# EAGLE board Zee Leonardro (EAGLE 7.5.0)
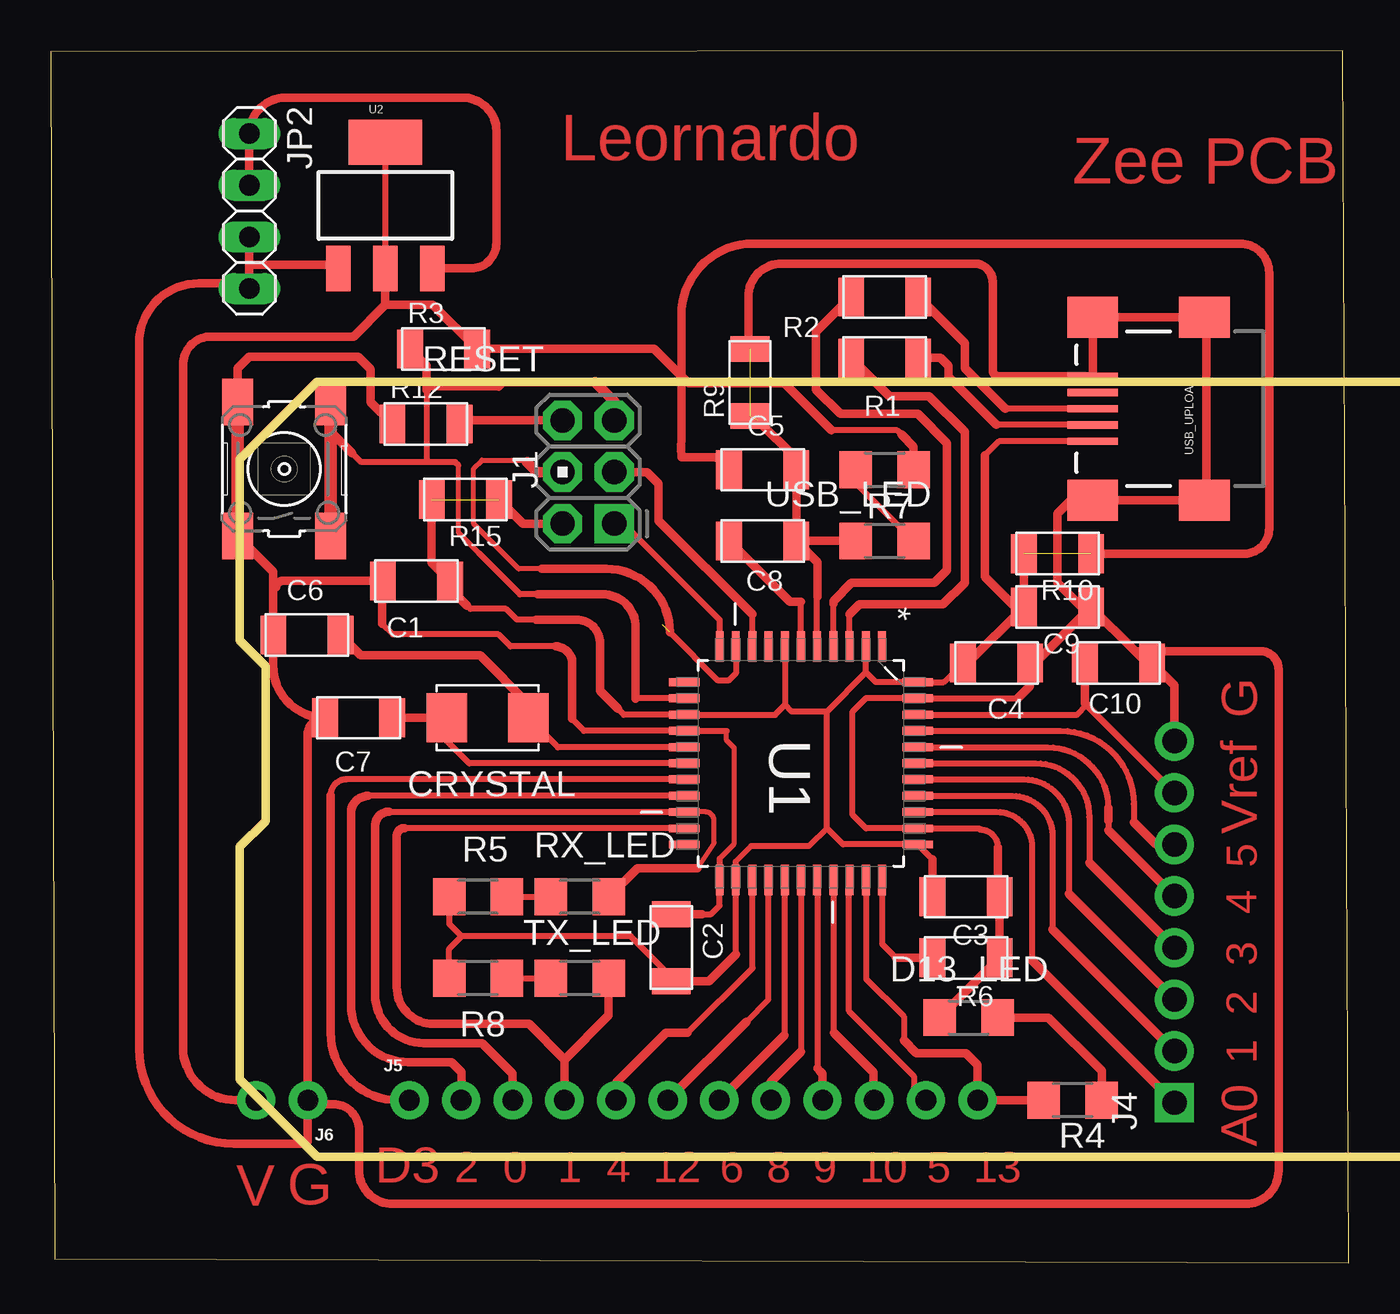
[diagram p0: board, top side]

Size 63.84 x 59.6 mm. Coordinates in mm from the lower left corner, seen from the top.
Outline: 0.19,0.21 63.84,0 63.56,59.6 0,59.57 0.19,0.21
Copper layers (1*16): Top 0.035mm / dielectric 1.5mm / Bottom 0.035mm
Design rules "default *": minimum track width 10mil, minimum drill 24mil, track to track 0.4mm, track to pad 0.4mm, pad to pad 0.4mm, via to via 0.4mm, smd to smd 0.4mm, copper to edge 40mil, drill to drill 0.4mm, minimum pad ring 10mil, minimum via ring 8mil, stop-mask expansion 4mil, vias tented up to drill 0mil, thermal gap 10mil
Net classes: 0 default: width 0.305 mm, drill 0.305 mm, clearance 0.305 mm
Milling: area 9.3,5.2 to 109.6,43.3

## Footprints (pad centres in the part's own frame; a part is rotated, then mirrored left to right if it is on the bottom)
C1206FAB = smd 1.27 x 1.905: 1 -1.651,0; 2 1.651,0
2-SMD-5X3MM = smd 2 x 2.4: P$1 -2,0; P$2 2,0
1206 = smd 1.6 x 1.803: 1 -1.422,0; 2 1.422,0
2X3-NS = drill 1.2 pad 1.93 square: 1 -2.54,-1.27 | drill 1.2 pad 1.93 octagon: 2 -2.54,1.27; 3 0,-1.27; 4 0,1.27; 5 2.54,-1.27; 6 2.54,1.27
1X08_PIN1_NO_SILK = drill 1.2 pad 1.93 square: 1 0,0 | drill 1.2 pad 1.93: 2 2.54,0; 3 5.08,0; 4 7.62,0; 5 10.16,0; 6 12.7,0; 7 15.24,0; 8 17.78,0
1X12_NO_SILK = drill 1.016 pad 1.88: 1 0,0; 2 2.54,0; 3 5.08,0; 4 7.62,0; 5 10.16,0; 6 12.7,0; 7 15.24,0; 8 17.78,0; 9 20.32,0; 10 22.86,0; 11 25.4,0; 12 27.94,0
1X02_NO_SILK = drill 1.016 pad 1.88: 1 0,0; 2 2.54,0
1X04 = drill 1.016 long: 1 -3.81,0; 2 -1.27,0; 3 1.27,0; 4 3.81,0
R1206FAB = smd 1.27 x 1.905: 1 -1.651,0; 2 1.651,0
6MM_SWITCH = smd 2.286 x 1.524: 1 -3.302,2.286; 2 3.302,2.286; 3 -3.302,-2.286; 4 3.302,-2.286
QFP80P1200X1200X120-44N = smd 1.5 x 0.38: 1 -5.74,3.988; 2 -5.74,3.2; 3 -5.74,2.388; 4 -5.74,1.6; 5 -5.74,0.787; 6 -5.74,0; 7 -5.74,-0.787; 8 -5.74,-1.6; 9 -5.74,-2.388; 10 -5.74,-3.2; 11 -5.74,-3.988; 23 5.74,-3.988; 24 5.74,-3.2; 25 5.74,-2.388; 26 5.74,-1.6; 27 5.74,-0.787; 28 5.74,0; 29 5.74,0.787; 30 5.74,1.6; 31 5.74,2.388; 32 5.74,3.2; 33 5.74,3.988 | smd 0.38 x 1.5: 12 -3.988,-5.74; 13 -3.2,-5.74; 14 -2.388,-5.74; 15 -1.6,-5.74; 16 -0.787,-5.74; 17 0,-5.74; 18 0.787,-5.74; 19 1.6,-5.74; 20 2.388,-5.74; 21 3.2,-5.74; 22 3.988,-5.74; 34 3.988,5.74; 35 3.2,5.74; 36 2.388,5.74; 37 1.6,5.74; 38 0.787,5.74; 39 0,5.74; 40 -0.787,5.74; 41 -1.6,5.74; 42 -2.388,5.74; 43 -3.2,5.74; 44 -3.988,5.74
SOT223 = smd 1.219 x 2.235: 1 -2.311,-3.099; 2 0,-3.099; 3 2.311,-3.099 | smd 3.6 x 2.2: 4 0,3.099
USB_MINIB = smd 2.5 x 0.35: D+ 3.77,0; D- 3.77,0.8; GND 3.77,-1.6; ID 3.77,-0.8; VBUS 3.77,1.6 | smd 2.5 x 2: SHIELD@1 -1.73,-4.5; SHIELD@2 -1.73,4.5; SHIELD@3 3.77,4.5; SHIELD@4 3.77,-4.5

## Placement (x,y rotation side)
C1  0.1uF  [C1206FAB]  17.98,33.54 180 top
C2  0.1uF  [C1206FAB]  30.52,15.5 90 top
C3  0.1uF  [C1206FAB]  45.02,18 0 top
C4  0.1uF  [C1206FAB]  46.52,29.5 0 top
C5  0.1uF  [C1206FAB]  35.02,39 0 top
C6  18pF  [C1206FAB]  12.6,30.87 180 top
C7  18pF  [C1206FAB]  15.14,26.81 180 top
C8  0.1uF  [C1206FAB]  35.02,35.5 0 top
C9  0.1uF  [C1206FAB]  49.52,32.25 0 top
C10  0.1uF  [C1206FAB]  52.52,29.5 0 top
CRYSTAL  CRYSTAL  [2-SMD-5X3MM]  21.49,26.81 0 top
D13_LED  [1206]  45.14,12.06 180 top
J1  AVR_SPI_PRG_6NS  [2X3-NS]  26.44,38.89 90 top
J4  [1X08_PIN1_NO_SILK]  55.27,7.88 90 top
J5  [1X12_NO_SILK]  17.64,8 0 top
J6  [1X02_NO_SILK]  12.64,8 180 top
JP2  [1X04]  9.77,51.72 270 top
R1  22  [R1206FAB]  41.02,44.5 0 top
R2  22  [R1206FAB]  41.02,47.5 0 top
R3  10K  [R1206FAB]  19.32,44.94 0 top
R4  499  [1206]  50.27,8 0 top
R5  499  [1206]  21.02,18 0 top
R6  680  [R1206FAB]  45.02,15 0 top
R7  499  [1206]  41.02,39 180 top
R8  499  [1206]  21.02,14 0 top
R9  0  [R1206FAB]  34.39,43.29 90 top
R10  0  [R1206FAB]  49.52,34.88 180 top
R12  0  [R1206FAB]  18.45,41.25 0 top
R15  0  [R1206FAB]  20.39,37.53 180 top
RESET  [6MM_SWITCH]  11.48,39.04 90 top
RX_LED  [1206]  26.02,18 0 top
TX_LED  [1206]  26.02,14 0 top
U1  ATMEGA32U4-AU  [QFP80P1200X1200X120-44N]  36.9,24.57 270 top
U2  [SOT223]  16.45,52 0 top
USB_LED  [1206]  41.02,35.5 180 top
USB_UPLOAD  USB_MINIB  [USB_MINIB]  55.02,42 180 top

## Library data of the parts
C1-C10 CRYSTAL R1-R3 R6 R9 R10 R12 R15 RESET USB_UPLOAD = fab
D13_LED R4 R5 R7 R8 RX_LED TX_LED USB_LED = ng
J1 J4 = SparkFun-ConnectorsModified
J5 J6 = SparkFun-Connectors
JP2 = pinhead
U1 = Atmel_By_element14_Batch_1; MPN: ATMEGA32U4-AU; OC_FARNELL: 1748525; OC_NEWARK: 26R5633; PACKAGE: TQFP-44; SUPPLIER: Atmel
U2 = fab; PROD_ID: VREG-08170

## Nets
12V: JP2.1 JP2.2 U2.3
A0: J4.1 U1.36
A1: J4.2 U1.37
A2: J4.3 U1.38
A3: J4.4 U1.39
A4: J4.5 U1.40
A5: J4.6 U1.41
AREF: C10.1 J4.7 U1.42
D0: J5.3 RX_LED.2 U1.20
D1: J5.4 TX_LED.2 U1.21
D2: J5.2 U1.19
D3: J5.1 U1.18
D4: J5.5 U1.25
D5: J5.11 U1.31
D6: J5.7 U1.27
D7: U1.1
D8: J5.8 U1.28
D9: J5.9 U1.29
D10: J5.10 U1.30
D11: U1.12
D12: J5.6 U1.26
D13: J5.12 R4.1 U1.32
D14: U1.8
D15: J1.3 U1.9
D16: J1.4 U1.10
D17: J1.1 U1.11
D+: R2.1 U1.4
D-: R1.1 U1.3
GND: C1.2 C2.2 C3.2 C4.2 C5.2 C6.2 C7.2 C8.2 C9.2 C10.2 D13_LED.2 J4.8 J6.1 JP2.3 JP2.4 R6.2 R9.1 R9.2 R12.1 RESET.1 RESET.2 U1.5 U1.15 U1.23 U1.35 U1.43 U2.1 USB_LED.2 USB_UPLOAD.GND USB_UPLOAD.SHIELD@1 USB_UPLOAD.SHIELD@2 USB_UPLOAD.SHIELD@3 USB_UPLOAD.SHIELD@4
N$1: R1.2 USB_UPLOAD.D-
N$2: R2.2 USB_UPLOAD.D+
N$3: D13_LED.1 R4.2
N$4: R5.2 RX_LED.1
N$5: R7.2 USB_LED.1
N$6: R8.2 TX_LED.1
N$13: J1.6 R12.2
N$35: R6.1 U1.33
RESET: J1.5 R3.1 RESET.3 RESET.4 U1.13
TXLED: U1.22
UCAP: C8.1 U1.6
VCC: C1.1 C2.1 C3.1 C4.1 C5.1 C9.1 J1.2 J6.2 R3.2 R5.1 R7.1 R8.1 R10.1 R10.2 R15.1 R15.2 U1.2 U1.7 U1.14 U1.24 U1.34 U1.44 U2.2 U2.4 USB_UPLOAD.VBUS
XTAL1: C7.1 CRYSTAL.P$1 U1.17
XTAL2: C6.1 CRYSTAL.P$2 U1.16

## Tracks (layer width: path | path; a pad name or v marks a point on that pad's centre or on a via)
12V
  Top 0.406: JP2.2 JP2.1 arc-90 11.52,57.29 19.53,57.29 20.29,57.29 | 20.29,57.29 20.55,57.29 | U2.3 arc90 18.57,48.7 18.57,48.37 arc-90 19.1,48.91 20.67,48.91 arc90 21.92,50.15 21.92,55.66 arc90 20.29,57.29
A0
  Top 0.305: U1.36 46.53,22.18 arc-90 48.27,20.44 48.27,14.88
  Top 0.406: 48.27,14.88 J4.1
A1
  Top 0.305: U1.37 47.3,22.97 arc-90 49.27,21 49.27,16.42
  Top 0.406: 49.27,16.42 J4.2
A2
  Top 0.305: U1.38 47.86,23.78 arc-90 50.08,21.56 50.08,18.14
  Top 0.406: 50.08,18.14 J4.3
A3
  Top 0.305: U1.39 48.45,24.57 arc-90 51.08,21.94 51.08,19.68
  Top 0.406: 51.08,19.68 J4.4
A4
  Top 0.305: U1.40 49.04,25.35 arc-90 52.02,22.38 | 52.02,21.75 52.02,21.29
  Top 0.406: 52.02,21.29 J4.5 | 52.02,22.38 52.02,21.75
A5
  Top 0.305: U1.41 49.68,26.17 arc-90 53.27,22.58 53.27,21.66
  Top 0.406: 53.27,21.66 54.35,20.58 J4.6
AREF
  Top 0.305: U1.42 50.47,26.95 50.95,27.43
  Top 0.356: 50.95,27.43 J4.7
  Top 0.406: 50.95,27.43 50.86,27.52 C10.1
D0
  Top 0.254: 31.8,19.42 32.64,20.66 arc-90 32.61,20.69 32.61,21.78 arc90 32.21,22.18 U1.20
  Top 0.305: 16.64,22.19 U1.20
  Top 0.406: 22.77,8 J5.3 22.7,8.02 22.7,9.31 21.2,10.81 18.33,10.81 arc-90 15.95,13.19 15.95,21.5 arc-90 16.64,22.19 | RX_LED.2 28.85,19.42 31.8,19.42
D1
  Top 0.305: 17.39,21.38 17.4,21.37 U1.21
  Top 0.406: 25.27,10 23.52,11.75 19.33,11.75 18.83,11.75 arc-90 17.02,13.56 17.02,21 arc-90 17.39,21.38 | 25.27,10 J5.4 | TX_LED.2 27.44,12.17 25.27,10
D2
  Top 0.305: U1.19 15.61,22.97
  Top 0.406: J5.2 20.2,8.02 20.2,9.38 19.7,9.88 18.08,9.88 17.58,9.88 arc-90 14.77,12.69 14.77,22.13 arc-90 15.61,22.97
D3
  Top 0.305: U1.18 14.54,23.78 arc90 13.77,23
  Top 0.406: 13.77,23 13.77,11.88 arc90 13.76,11.88 13.76,11.31 arc90 17.08,8 J5.1
D4
  Top 0.305: U1.25 34.52,14.5 31.33,11.31
  Top 0.406: J5.5 27.8,8.85 30.27,11.31 31.33,11.31
D5
  Top 0.305: U1.31 39.27,18.81 39.27,12.38 42.45,9.19 42.45,8.59 J5.11
D6
  Top 0.305: U1.27 36.08,18.8 36.08,11.19
  Top 0.406: J5.7 35.5,10.61 36.08,11.19
D8
  Top 0.305: 36.89,10.38 36.9,10.38 U1.28
  Top 0.406: 36.89,10.38 35.39,8.88 35.39,8.03 J5.8
D9
  Top 0.305: U1.29 37.7,18.81 37.7,9.56
  Top 0.406: J5.9 37.96,9.31 37.84,9.42 37.7,9.56
D10
  Top 0.305: 38.78,11.05 38.5,11.33 U1.30
  Top 0.406: 38.52,11.31 38.78,11.05 40.45,9.38 40.45,8.05 J5.10
D12
  Top 0.305: U1.26 35.3,12.96 34.21,11.87
  Top 0.406: J5.6 34.21,11.87
D13
  Top 0.305: 41.95,10.94 41.95,12.13 40.1,13.98 U1.32
  Top 0.406: R4.1 J5.12 45.58,9.75 45.02,10.31 42.58,10.31 41.95,10.94
D15
  Top 0.305: U1.9 34.51,31.88
  Top 0.406: J1.3 29.32,38.89 29.89,38.31 29.89,36.5 34.51,31.88
D16  (1 unrouted)
  Top 0.254: 24.14,34.13 23.02,34.13 20.8,36.35 20.8,39.06 21.2,39.47 23.33,39.47 23.42,39.38 23.55,39.25
  Top 0.305: U1.10 33.7,28.99 33.33,28.63 32.83,28.63 30.45,31
  Top 0.406: 24.14,34.13 27.33,34.13 arc-90 30.45,31
  Top 0.508: J1.4 23.91,38.89 23.42,39.38
D17
  Top 0.305: U1.11 32.91,31.61 28.17,36.35 J1.1
D+
  Top 0.305: U1.4 38.5,32.42
  Top 0.406: 38.5,32.42 38.5,32.54 39.39,33.44 43.45,33.44 44.08,34.06 44.08,40.31 42.64,41.75 38.83,41.75 37.64,42.94 37.64,45.78 R2.1
D-
  Top 0.305: U1.3 39.28,31.89
  Top 0.406: R1.1 41.24,42.63 43.2,42.63 44.95,40.88 44.95,33.44 43.89,32.38 39.77,32.38 39.28,31.89
GND  (2 unrouted)
  Top 0.254: 32.91,19.89 33.63,20.61 33.63,25.31 33.24,25.69 33.24,26.15
  Top 0.305: U1.5 37.68,32.73 37.7,32.75 | 25.64,26.75 26.23,26.17 U1.15 33.24,26.17 33.24,26.15 | RESET.1 9.71,35.22 | 47.58,27.77 U1.43 40.1,27.77 39.44,27.11 39.44,22.03 40.1,21.37 U1.35 45.65,21.37 45.7,21.31 arc-90 46.58,20.44 | 32.04,17.15 32.48,17.15 32.89,17.56 32.89,18.81 U1.23 32.91,19.89 | 24.83,30.31 22.61,30.31 22.02,30.91 16.83,30.91 16.3,31.44 | 50.86,32.1 50.67,32.28
  Top 0.406: 46.58,20.44 46.58,18.09 C3.2 R6.2 D13_LED.2 | 56.58,37.5 USB_UPLOAD.SHIELD@3 50.17,37.5 49.52,36.85 49.52,33.44 50.67,32.28 50.93,32.02 | 56.58,37.5 USB_UPLOAD.SHIELD@2 | RESET.2 9.19,44 9.76,44.56 15.11,44.56 15.73,43.94 15.73,42.32 R12.1 | C2.2 32.04,17.15 | 37.7,32.75 37.7,34.47 C8.2 | C8.2 USB_LED.2 | C8.2 C5.2 36.67,39.54 34.77,41.44 | 25.64,26.75 25.64,29.5 arc90 24.83,30.31 | J4.8 55.27,28.4 C10.2 53.92,29.5 53.33,30.09 | 53.33,30.09 C9.2 50.93,32.02 | 50.93,32.02 48.42,29.5 C4.2 48.17,28.36 47.58,27.77 | 12.7,7.94 J6.1 | 56.58,37.5 56.83,37.75 56.83,46.42 USB_UPLOAD.SHIELD@1 USB_UPLOAD.SHIELD@4 USB_UPLOAD.GND 46.63,43.6 arc-90 46.33,43.9 46.33,48.25 arc90 45.44,49.14 35.94,49.14 arc90 34.31,47.51 34.31,45.02 arc90 R9.2 34.83,44.94 | 16.3,31.44 16.3,33.5 C1.2 11.4,33.54 arc90 11.08,33.22 10.95,33.22 | J6.1 12.99,7.66 arc-90 13.14,7.81 13.89,7.81 arc-90 15.16,6.54 15.16,4.56 arc90 16.81,2.91 58.77,2.91 arc90 60.39,4.53 60.39,29.18 arc90 59.48,30.09 53.33,30.09 | 10.95,33.22 C6.2 10.95,29.35 arc90 C7.2 C7.2 arc90 12.64,25.96 J6.1 | 10.95,33.22 10.95,33.99 9.71,35.22 | 9.77,49.08 JP2.4 arc90 9.51,48.17 7.29,48.17 arc90 4.34,45.22 4.34,10.53 arc90 9.02,5.85 12.44,5.85 arc90 12.64,6.05 J6.1 | 9.77,49.08 JP2.3 | U2.1 14.14,49.08 9.77,49.08
  Top 0.61: RESET.1 RESET.2
N$1
  Top 0.305: USB_UPLOAD.D- 46.5,41.2
  Top 0.406: 46.5,41.2 44.14,43.56 44.14,44.13 43.77,44.5 R1.2
N$2
  Top 0.305: USB_UPLOAD.D+ 46.95,42
  Top 0.406: 46.95,42 44.95,44 44.95,45.22 R2.2
N$3
  Top 0.406: R4.2 51.69,9.46 49.08,12.06 D13_LED.1
N$4
  Top 0.305: R5.2 RX_LED.1
N$5
  Top 0.305: R7.2 39.59,38.35 USB_LED.1
N$6
  Top 0.305: R8.2 TX_LED.1
N$13
  Top 0.406: R12.2 20.29,41.44 25.16,41.44
  Top 0.508: 25.16,41.44 J1.6
N$35
  Top 0.305: U1.33 40.88,16.28 40.88,15.88 40.88,15.7 41.58,15
  Top 0.406: 41.58,15 R6.1
RESET
  Top 0.254: 21.05,34.91 20.05,35.91 20.05,39.22
  Top 0.305: U1.13 28.78,27.77 28.77,27.75 | 23.95,32.88 23.08,32.88 21.05,34.91 | 20.05,39.22 19.89,39.38 18.48,39.38 | 18.48,39.38 15.27,39.38 14.83,39.81 | 18.48,42.91 18.48,39.38 | 22.33,43.31 22.05,43.03 18.55,43.03 18.48,43.1
  Top 0.406: RESET.4 13.76,40.88 14.83,39.81 | 28.77,27.75 28.77,31.25 arc90 27.14,32.88 23.95,32.88 | 26.77,43.31 22.33,43.31 | R3.1 18.48,44.12 18.48,43.1 18.48,42.91
  Top 0.508: J1.5 27.71,42.37 26.77,43.31
  Top 0.61: RESET.4 RESET.3
UCAP
  Top 0.305: U1.6 36.9,32.5 36.89,32.5
  Top 0.406: 36.89,32.5 36.36,32.5 C8.1
VCC  (2 unrouted)
  Top 0.254: 33.7,19.74 34.45,20.5
  Top 0.305: 38.17,21.38 38.17,27.11 | U1.7 36.11,27.44 | 40.1,29.04 40.58,28.56 U1.44 43.92,28.56 C4.1 | 40.1,29.04 38.17,27.11 | 36.11,27.44 35.62,26.95 U1.14 28.19,26.95 27.89,27.25 | 38.17,27.11 36.44,27.11 36.11,27.44 | 38.17,21.38 38.96,20.58 U1.34 43.36,19.85 | 38.17,21.38 37.29,20.5 34.45,20.5 | 40.1,29.04 U1.2 | 33.7,15.19 U1.24 33.7,19.74 | C2.1 30.52,14.06 28.52,16.06 20.2,16.06 | R5.1 19.59,16.67 20.2,16.06 | R8.1 19.59,15.46 20.2,16.06 | 41.83,40.75 41.64,40.94 38.39,40.94 | USB_UPLOAD.VBUS 46.64,40.4 45.95,39.71 | 20.48,32.31 20.64,32.16 22.39,32.16 22.92,31.63 23.86,31.63 24.02,31.63 | U2.4 U2.2
  Top 0.406: C2.1 32.36,13.85 33.7,15.19 | R7.1 42.44,40.14 41.83,40.75 | 38.39,40.94 36.08,43.25 31.36,43.25 31.02,43.6 | C4.1 45.11,29.5 C9.1 | 47.79,32.33 C9.1 | C9.1 48.02,32.4 47.86,32.55 R10.2 | 10.2,8 J6.2 9.1,8 arc-90 6.5,10.6 6.5,44.16 arc-90 7.9,45.55 14.88,45.55 16.45,47.12 | C9.1 47.45,32.25 45.95,33.75 45.95,39.71 | C3.1 43.36,19.85 | C1.1 | 20.48,32.31 19.64,33.16 C1.1 | R15.1 23.23,36.35 J1.2 | R15.2 18.74,34.43 C1.1 | 31.02,43.6 31.02,40.58 30.99,40.09 31.02,39.63 32.53,39.63 arc-90 33.26,38.9 arc90 C5.1 | 31.02,43.6 29.67,44.94 R3.2 18.79,47.12 16.45,47.12 | 27.89,27.25 27.02,28.13 27.02,30.47 arc90 25.86,31.63 23.86,31.63 | 16.45,47.12 U2.2 | 31.02,43.6 arc-90 31.01,43.6 31.01,46.6 arc-90 34.54,50.13 58.49,50.13 arc-90 59.92,48.7 59.92,36.1 arc-90 58.7,34.88 R10.1
XTAL1
  Top 0.305: U1.17 20.58,24.57 19.49,25.66 CRYSTAL.P$1
  Top 0.406: C7.1 CRYSTAL.P$1
XTAL2
  Top 0.305: CRYSTAL.P$2 24.94,25.35 U1.16
  Top 0.406: C6.1 15.24,29.88 21.11,29.88 23.49,27.5 CRYSTAL.P$2

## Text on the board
Top: Leornardo | Zee PCB | G | Vref | 5 | 4 | 3 | 2 | 1 | A0 | D3 | 2 | 0 | 1 | 4 | 12 | 6 | 8 | 9 | 10 | 5 | 13 | V | G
